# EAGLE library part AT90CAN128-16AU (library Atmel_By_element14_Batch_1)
CAN Controller
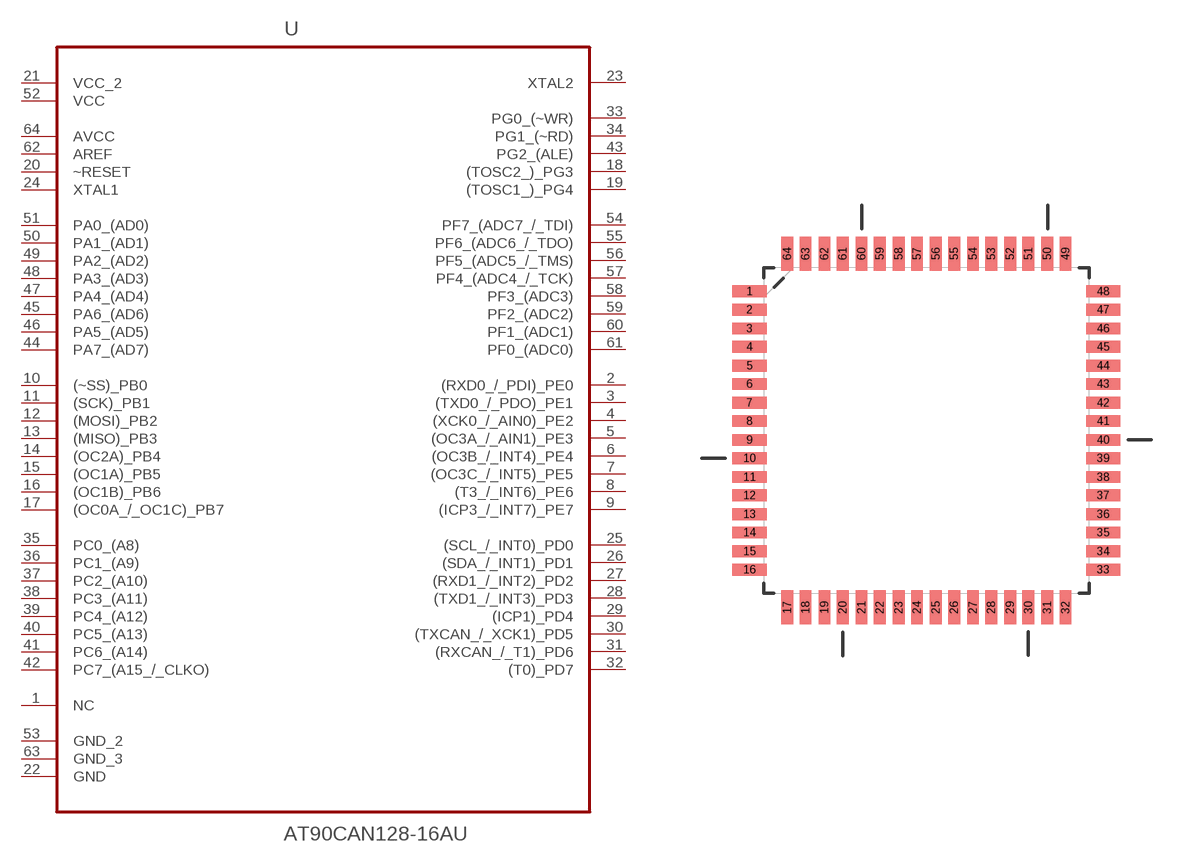
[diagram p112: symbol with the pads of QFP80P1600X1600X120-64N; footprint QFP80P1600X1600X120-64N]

Designator prefix U

## AT90CAN128-16AU (MPN: AT90CAN128-16AU; OC_FARNELL: 1455065; OC_NEWARK: 58M3860; PACKAGE: TQFP-64; SUPPLIER: Atmel)  [QFP80P1600X1600X120-64N]
1  NC  nc
2  (RXD0_/_PDI)_PE0
3  (TXD0_/_PDO)_PE1
4  (XCK0_/_AIN0)_PE2
5  (OC3A_/_AIN1)_PE3
6  (OC3B_/_INT4)_PE4
7  (OC3C_/_INT5)_PE5
8  (T3_/_INT6)_PE6
9  (ICP3_/_INT7)_PE7
10  (~SS)_PB0
11  (SCK)_PB1
12  (MOSI)_PB2
13  (MISO)_PB3
14  (OC2A)_PB4
15  (OC1A)_PB5
16  (OC1B)_PB6
17  (OC0A_/_OC1C)_PB7
18  (TOSC2_)_PG3
19  (TOSC1_)_PG4
20  ~RESET  in
21  VCC_2  pwr
22  GND  pas
23  XTAL2  out
24  XTAL1  in
25  (SCL_/_INT0)_PD0
26  (SDA_/_INT1)_PD1
27  (RXD1_/_INT2)_PD2
28  (TXD1_/_INT3)_PD3
29  (ICP1)_PD4
30  (TXCAN_/_XCK1)_PD5
31  (RXCAN_/_T1)_PD6
32  (T0)_PD7
33  PG0_(~WR)
34  PG1_(~RD)
35  PC0_(A8)
36  PC1_(A9)
37  PC2_(A10)
38  PC3_(A11)
39  PC4_(A12)
40  PC5_(A13)
41  PC6_(A14)
42  PC7_(A15_/_CLKO)
43  PG2_(ALE)
44  PA7_(AD7)
45  PA6_(AD6)
46  PA5_(AD5)
47  PA4_(AD4)
48  PA3_(AD3)
49  PA2_(AD2)
50  PA1_(AD1)
51  PA0_(AD0)
52  VCC  pwr
53  GND_2  pas
54  PF7_(ADC7_/_TDI)
55  PF6_(ADC6_/_TDO)
56  PF5_(ADC5_/_TMS)
57  PF4_(ADC4_/_TCK)
58  PF3_(ADC3)
59  PF2_(ADC2)
60  PF1_(ADC1)
61  PF0_(ADC0)
62  AREF  in
63  GND_3  pas
64  AVCC  pwr

## Footprint QFP80P1600X1600X120-64N (pad centres in mm)
smd 1.473 x 0.508: 1 -7.62,5.994; 2 -7.62,5.207; 3 -7.62,4.394; 4 -7.62,3.607; 5 -7.62,2.794; 6 -7.62,2.007; 7 -7.62,1.194; 8 -7.62,0.406; 9 -7.62,-0.406; 10 -7.62,-1.194; 11 -7.62,-2.007; 12 -7.62,-2.794; 13 -7.62,-3.607; 14 -7.62,-4.394; 15 -7.62,-5.207; 16 -7.62,-5.994; 33 7.62,-5.994; 34 7.62,-5.207; 35 7.62,-4.394; 36 7.62,-3.607; 37 7.62,-2.794; 38 7.62,-2.007; 39 7.62,-1.194; 40 7.62,-0.406; 41 7.62,0.406; 42 7.62,1.194; 43 7.62,2.007; 44 7.62,2.794; 45 7.62,3.607; 46 7.62,4.394; 47 7.62,5.207; 48 7.62,5.994
smd 0.508 x 1.473: 17 -5.994,-7.62; 18 -5.207,-7.62; 19 -4.394,-7.62; 20 -3.607,-7.62; 21 -2.794,-7.62; 22 -2.007,-7.62; 23 -1.194,-7.62; 24 -0.406,-7.62; 25 0.406,-7.62; 26 1.194,-7.62; 27 2.007,-7.62; 28 2.794,-7.62; 29 3.607,-7.62; 30 4.394,-7.62; 31 5.207,-7.62; 32 5.994,-7.62; 49 5.994,7.62; 50 5.207,7.62; 51 4.394,7.62; 52 3.607,7.62; 53 2.794,7.62; 54 2.007,7.62; 55 1.194,7.62; 56 0.406,7.62; 57 -0.406,7.62; 58 -1.194,7.62; 59 -2.007,7.62; 60 -2.794,7.62; 61 -3.607,7.62; 62 -4.394,7.62; 63 -5.207,7.62; 64 -5.994,7.62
